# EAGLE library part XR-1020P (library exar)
Telecom instrumentation FILTER
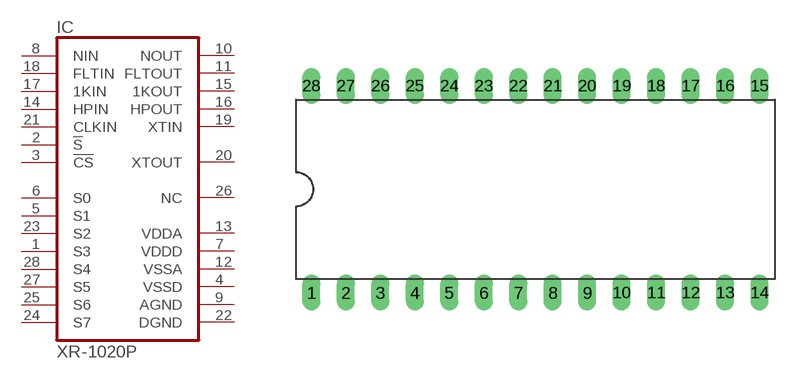
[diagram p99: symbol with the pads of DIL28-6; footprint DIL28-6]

Designator prefix IC

## XR-1020P (OC_FARNELL: unknown; OC_NEWARK: unknown)  [DIL28-6]
1  S3  in
2  !S  in
3  !CS  in
4  VSSD  pwr
5  S1  in
6  S0  in
7  VDDD  pwr
8  NIN  in
9  AGND  pwr
10  NOUT  out
11  FLTOUT  out
12  VSSA  pwr
13  VDDA  pwr
14  HPIN  in
15  1KOUT  out
16  HPOUT  out
17  1KIN  in
18  FLTIN  in
19  XTIN  in
20  XTOUT  out
21  CLKIN  in
22  DGND  pwr
23  S2  in
24  S7  in
25  S6  in
26  NC  nc
27  S5  in
28  S4  in

## Footprint DIL28-6 (pad centres in mm)
Dual In Line Package 0.6 inch
drill 0.813 long: 1 -16.51,-7.62; 2 -13.97,-7.62; 3 -11.43,-7.62; 4 -8.89,-7.62; 5 -6.35,-7.62; 6 -3.81,-7.62; 7 -1.27,-7.62; 8 1.27,-7.62; 9 3.81,-7.62; 10 6.35,-7.62; 11 8.89,-7.62; 12 11.43,-7.62; 13 13.97,-7.62; 14 16.51,-7.62; 15 16.51,7.62; 16 13.97,7.62; 17 11.43,7.62; 18 8.89,7.62; 19 6.35,7.62; 20 3.81,7.62; 21 1.27,7.62; 22 -1.27,7.62; 23 -3.81,7.62; 24 -6.35,7.62; 25 -8.89,7.62; 26 -11.43,7.62; 27 -13.97,7.62; 28 -16.51,7.62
